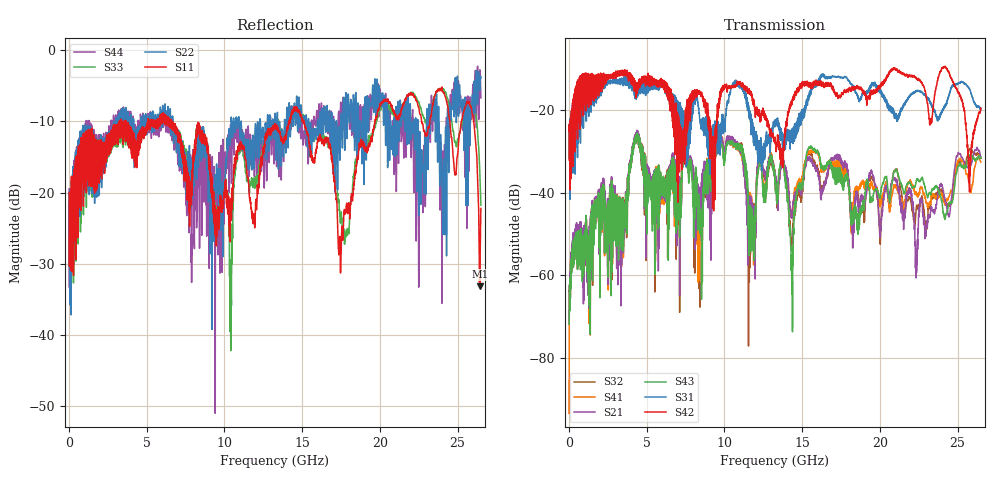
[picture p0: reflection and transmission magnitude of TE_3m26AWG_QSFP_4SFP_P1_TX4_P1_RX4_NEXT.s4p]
!Agilent Technologies,N5222A,MY51421691,A.10.00.00
!Agilent N5222A: A.10.00.00
!Date: Friday, January 30, 2015 12:35:01
!Correction: S11(Full 4 Port(1,2,3,4))
!S12(Full 4 Port(1,2,3,4))
!S13(Full 4 Port(1,2,3,4))
!S14(Full 4 Port(1,2,3,4))
!S21(Full 4 Port(1,2,3,4))
!S22(Full 4 Port(1,2,3,4))
!S23(Full 4 Port(1,2,3,4))
!S24(Full 4 Port(1,2,3,4))
!S31(Full 4 Port(1,2,3,4))
!S32(Full 4 Port(1,2,3,4))
!S33(Full 4 Port(1,2,3,4))
!S34(Full 4 Port(1,2,3,4))
!S41(Full 4 Port(1,2,3,4))
!S42(Full 4 Port(1,2,3,4))
!S43(Full 4 Port(1,2,3,4))
!S44(Full 4 Port(1,2,3,4))
!S4P File: Measurements: <S11,S12,S13,S14>,
!<S21,S22,S23,S24>,
!<S31,S32,S33,S34>,
!<S41,S42,S43,S44>:
# Hz S  dB  R 50.0
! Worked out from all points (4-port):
!   2650 points, 10 MHz to 26.5 GHz, reference 50 ohm
!   strongest paths, dB at 10 MHz, 6.63 GHz, 13.26 GHz, 19.88 GHz, 26.5 GHz:
!     S42: -25.0, -19.3, -27.0, -14.9, -19.5
!     S31: -24.8, -19.1, -23.3, -14.9, -19.7
!     S43: -72.0, -36.9, -37.3, -39.9, -31.6
!     S21: -71.3, -36.0, -35.8, -42.4, -31.6
!     S41: -93.5, -36.7, -35.8, -40.7, -32.6
!     S32: -63.9, -36.1, -37.2, -42.7, -31.5
!   lowest |S11| = -33.2 dB at 26.43 GHz (marker M1), VSWR 1.04, Z = 51.7 - j1.39 ohm
!   |S11| at or under -10 dB: start of sweep to 3.24 GHz; 6.606 GHz to 14.16 GHz (7.55 GHz wide, 72.7 % of centre); 15.11 GHz to 19.69 GHz (4.574 GHz wide, 26.3 % of centre)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
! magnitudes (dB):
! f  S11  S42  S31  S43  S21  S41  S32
! 10 MHz  -20.0  -25.0  -24.8  -72.0  -71.3  -93.5  -63.9
! 4.33 GHz  -14.7  -15.3  -17.3  -27.5  -27.2  -27.2  -27.6
! 14.33 GHz  -9.1  -18.1  -24.5  -58.8  -46.2  -45.3  -53.3
! 15.51 GHz  -13.3  -13.7  -15.3  -29.1  -31.6  -30.1  -30.3
! 22.35 GHz  -7.0  -12.1  -15.4  -37.0  -53.7  -39.9  -43.3
! 26.43 GHz  -33.2  -20.4  -19.4  -31.6  -30.3  -31.9  -30.7
! 26.5 GHz  -22.2  -19.5  -19.7  -31.6  -31.6  -32.6  -31.5
